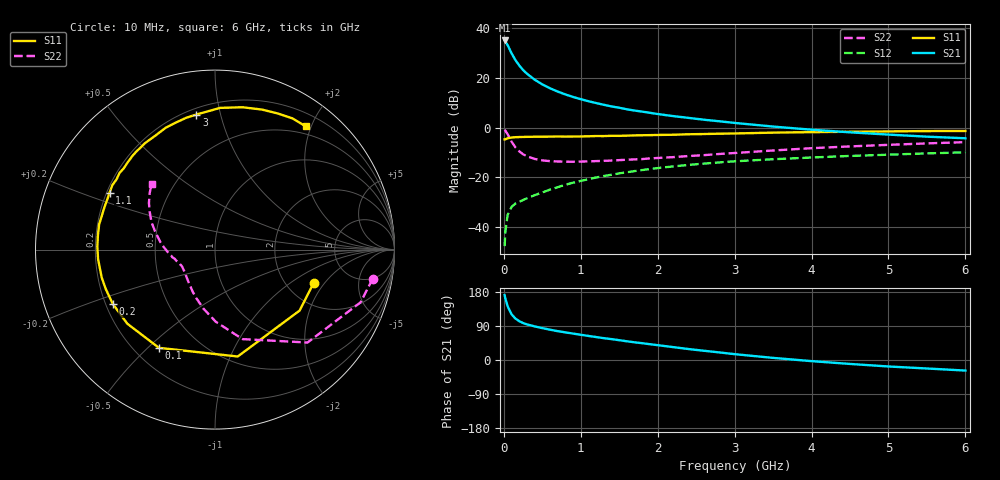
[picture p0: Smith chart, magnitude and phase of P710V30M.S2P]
! SIEMENS Small Signal Semiconductors
! BFP196
! Si NPN RF Bipolar Junction Transistor in SOT143
! VCE = 10 V  IC = 30 mA
! Common Emitter S-Parameters:  May  1996
# GHz  S  MA  R  50
!  f  S11  S21  S12  S22
! GHz  MAG  ANG  MAG  ANG  MAG  ANG  MAG  ANG
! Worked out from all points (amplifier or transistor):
!   36 points, 10 MHz to 6 GHz, reference 50 ohm
!   highest |S21| = 34.9 dB at 10 MHz (marker M1)
!   |S21| within 3 dB of that: start of sweep to 66.81 MHz
!   unconditionally stable (mu >= 1): 648.7 MHz to 4.502 GHz
!   at 250 MHz: K = 0.67, MSG = 26.0 dB, |S12| = -29.0 dB
!   at 1.4 GHz: K = 1.09, MAG = 11.8 dB, |S12| = -18.9 dB
!   at 6 GHz: K = 0.97, MSG = 2.8 dB, |S12| = -9.9 dB
!   S11 on the Smith chart (normalised r, x): 10 MHz: 2.79, -1.57; 100 MHz: 0.30, -0.54; 200 MHz: 0.23, -0.24; 1.1 GHz: 0.21, +0.24; 3 GHz: 0.24, +0.84; 6 GHz: 0.38, +1.92
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0.01  0.5802 -18.7  55.46 171.1  0.0042 75.3  0.8939 -10.4
0.02  0.581 -35.8  52.63 162.0  0.0083 72.0  0.8626 -19.9
0.05  0.609 -78.0  44.36 141.6  0.0179 57.5  0.7308 -45.1
0.1  0.6301 -119.7  30.85 120.7  0.0256 46.7  0.5219 -72.9
0.15  0.6396 -139.8  22.45 109.4  0.03 42.9  0.4019 -89.4
0.2  0.6449 -152.0  17.55 102.5  0.0325 43.3  0.334 -101.3
0.25  0.647 -160.2  14.2 97.6  0.0353 44.1  0.2907 -110.8
0.3  0.6501 -166.1  11.97 94.0  0.0382 46.6  0.2664 -117.6
0.4  0.6537 -175.5  9.11 88.7  0.0441 49.2  0.2349 -128.6
0.5  0.6557 178.6  7.299 84.2  0.05 52.1  0.2198 -136.4
0.6  0.6573 172.8  6.105 80.0  0.0571 53.7  0.2122 -141.7
0.7  0.6607 167.6  5.254 76.1  0.0637 54.6  0.2089 -146.0
0.9  0.6597 159.3  4.093 69.7  0.0785 55.3  0.2063 -152.5
1.1  0.6677 151.6  3.359 63.5  0.0922 54.9  0.2102 -156.8
1.3  0.6738 144.5  2.852 57.6  0.1068 53.5  0.215 -160.5
1.6  0.6877 135.0  2.317 49.4  0.1273 50.6  0.2264 -165.1
2.2  0.7165 117.7  1.694 34.0  0.1662 43.5  0.2552 -174.5
3  0.7596 97.8  1.236 15.4  0.2104 32.9  0.3086 171.8
3.5  0.7902 87.9  1.046 5.6  0.2317 26.4  0.3467 163.6
4.5  0.8228 71.5  0.801 -10.4  0.2695 15.1  0.4186 150.2
5.5  0.849 59.4  0.656 -22.4  0.3029 4.7  0.481 139.2
6  0.8526 53.6  0.609 -27.9  0.319 -0.9  0.5098 133.8
